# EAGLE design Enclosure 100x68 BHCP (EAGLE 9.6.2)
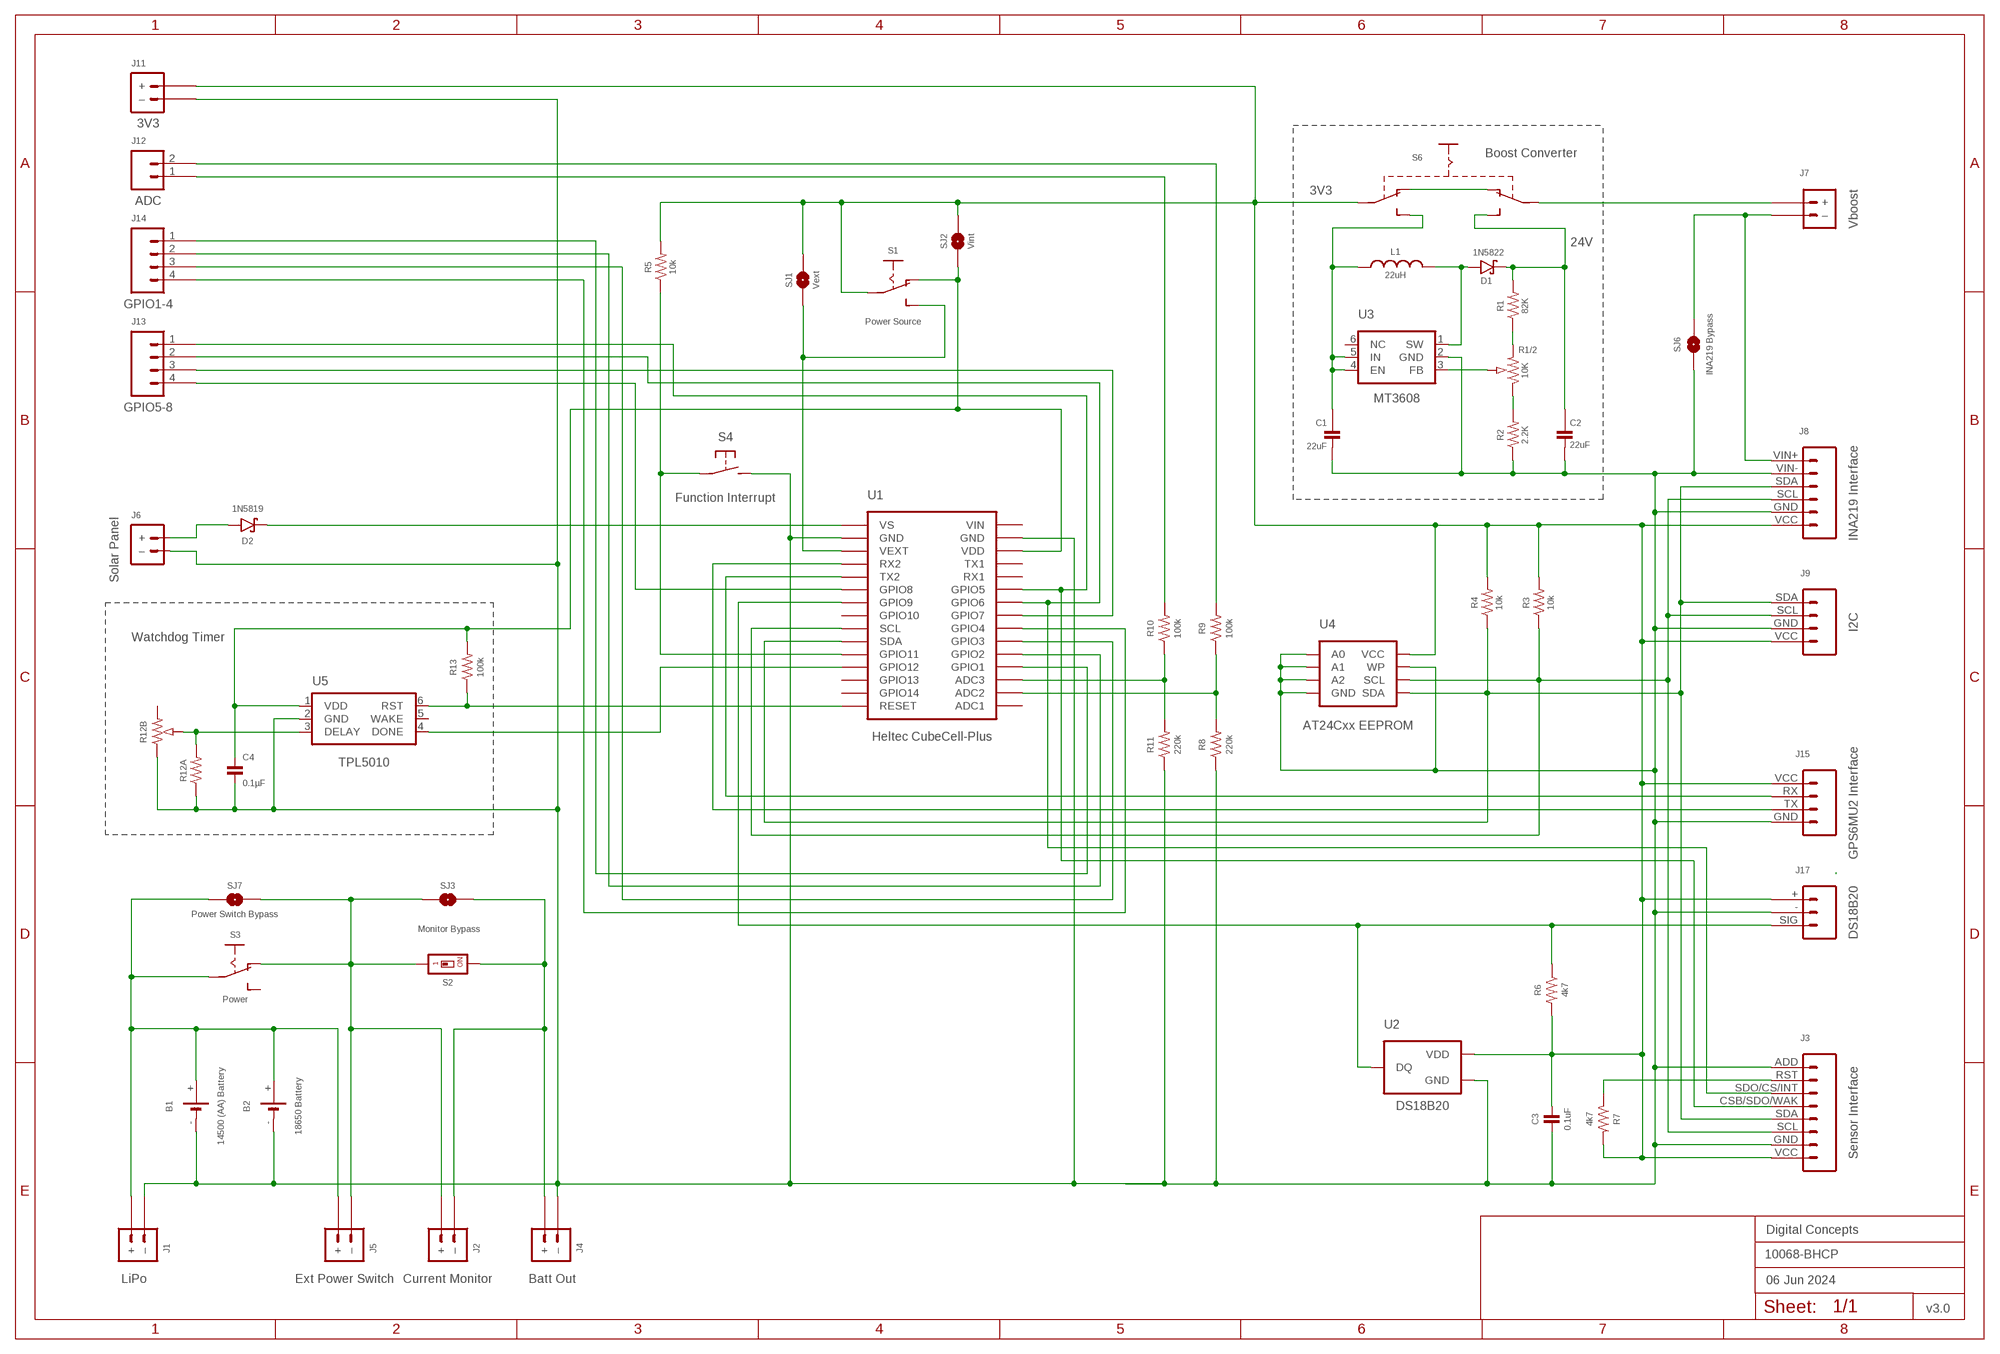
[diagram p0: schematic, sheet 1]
FRAME2 (A3L-LOC): DATE: 06 Jun 2024; OWNER: Digital Concepts; TITLE: 10068-BHCP; VERSION: v3.0

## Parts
B1  14500 (AA) Battery  BATTERY-HOLDER-14500(AA)  [BATTERY-14500]
B2  18650 Battery  BATTERY-HOLDER-18650  [BATTERY-18650]
C1  22uF  CAPACITOR-1206  [C1206]
C2  22uF  CAPACITOR-1206  [C1206]
C3  0.1uF  CAPACITOR-0805  [C0805]
C4  0.1µF  CAPACITOR-0805  [C0805]
D1  1N5822  DIODE-SCHOTTKY-1N5822  [DIODE_SMB]
D2  1N5819  1N5819-SOD-123  [SOD-123]
J1  LiPo  JST-PH2.0-2-H-POWER  [JST-PH2.0-2-HORIZONTAL-POWER]
J2  Current Monitor  JST-PH2.0-2-H-POWER  [JST-PH2.0-2-HORIZONTAL-POWER]
J3  Sensor Interface  HEADER-1X8-SENSOR  [CONN_08-SENSOR]
J4  Batt Out  JST-GH1.25-2-HORIZONTAL-POWER  [JST-GH1.25-2-HORIZONTAL]
J5  Ext Power Switch  JST-PH2.0-2-DUAL-POWER"  [JST-PH2.0-2-DUAL-POWER]
J6  Solar Panel  JST-PH2.0-2-VERTICAL  [JST-PH2.0-2-VERTICAL=POWER]
J7  Vboost  JST-PH2.0-2-H-POWER  [JST-PH2.0-2-HORIZONTAL-POWER]
J8  INA219 Interface  INA219-I2C-MODULE  [CONN_06-INA219]
J9  I2C  JST-PH2.0-I2C-MALE-HORIZONTAL  [JST-PH2.0-4-HORIZONTAL@1]
J11  3V3  JST-PH2.0-2-H-POWER  [JST-PH2.0-2-HORIZONTAL-POWER]
J12  ADC  JST-PH2.0-2-HORIZONTAL  [JST-PH2.0-2-HORIZONTAL]
J13  GPIO5-8  JST-PH2.0-4-HORIZONTAL  [JST-PH2.0-4-HORIZONTAL]
J14  GPIO1-4  JST-PH2.0-4-HORIZONTAL  [JST-PH2.0-4-HORIZONTAL]
J15  GPS6MU2 Interface  HEADER-1X4-GPS  [CONN_04-GPS]
J17  DS18B20  JST-PH2.0-3-HORIZONTAL-DS18B20  [JST-PH2.0-DS18B20-HORIZONTAL]
L1  22uH  INDUCTOR-CDRH104R/6D28L5038P  [CDRH104R+6D28]
R1  82K  RESISTORR0805  [R0805]
R1/2  10K  RESISTOR-TRIMM-BAOTER-H-US  [RTRIM64P]
R2  2.2K  RESISTORR0805  [R0805]
R3  10k  RESISTORR0805  [R0805]
R4  10k  RESISTORR0805  [R0805]
R5  10k  RESISTORR0805  [R0805]
R6  4k7  RESISTORR0805  [R0805]
R7  4k7  RESISTORR0805  [R0805]
R8  220k  RESISTORR0805  [R0805]
R9  100k  RESISTORR0805  [R0805]
R10  100k  RESISTORR0805  [R0805]
R11  220k  RESISTORR0805  [R0805]
R12A  RESISTORR0805  [R0805]
R12B  RESISTOR-TRIMM-33-US  [RTRIM3*3]
R13  100k  RESISTORR0805  [R0805]
S1  Power Source  SWITCH-SLIDE-SPDT-SMT  [SWITCH-SPDT-SMT]
S2  Monitor Bypass  SWITCH-DIP-SWS001  [SMD-001]
S3  Power  SWITCH-SLIDE-SPDT-PTH  [SWITCH-SPDT-PTH]
S4  Function Interrupt  SWITCH-MOMENTARY-2-PIN  [SWITCH-2-PAD]
S6  SWITCH-SLIDE-DPDT-PTH-S  [SWITCH-DPDT-PTH]
SJ1  Vext  SJ  [SJ]
SJ2  Vint  SJ-V-12  [SJ-VIA-12]
SJ3  Monitor  SJ  [SJ]
SJ6  INA219 Bypass  SJ  [SJ]
SJ7  Power Switch Bypass  SJ  [SJ]
U1  Heltec CubeCell-Plus  HELTEC-CUBECELL-PLUS-X  [HELTEC-CUBECELL=PLUS-X]
U2  DS18B20  THERMOMETER-DS18B20  [TO-92]
U3  MT3608  [SOT-23-6]
U4  AT24Cxx EEPROM  AT24CXX-EEPROM  [SOP-8]
U5  TPL5010  TPL5010DDCR  [SOT-23-6]

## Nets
GND: B1.- B2.- C1.2 C2.2 C3.2 C4.2 J1.-(–) J3.ADD J3.GND J4.-(–) J6.-(–) J8.GND J8.VIN- J9.GND J11.-(–) J15.GND J17.- R2.1 R8.1 R11.1 R12A.1 R12B.1(A) S4.P$2(S) SJ6.1 U1.GND@14(GND) U1.GND@17(GND) U2.1(GND) U3.2(GND) U4.P$1(A0) U4.P$2(A1) U4.P$3(A2) U4.P$4(GND) U4.P$7(WP) U5.2(GND)
N$1: D2.A J6.+
N$2: R10.1 R11.2 U1.ADC3
N$3: J2.-(–) J4.+ S2.2 SJ3.1
N$4: B1.+ B2.+ J1.+ J5.+ S3.2(P) SJ7.2
N$5: D2.C U1.VS
N$6: D1.A L1.1 U3.1(SW)
N$7: J12.1 R10.2
N$8: J3.SCL J8.SCL J9.SCL R3.1 U1.SCL U4.P$6(SCL)
N$9: J3.RST R7.1
N$10: J3.CSB/SDO/WAK J13.1 U1.GPIO5
N$11: J3.SDA J8.SDA J9.SDA R4.1 U1.SDA U4.P$5(SDA)
N$12: J13.4 U1.GPIO8
N$13: S1.3(S) SJ1.1 U1.VEXT
N$14: J15.RX U1.TX2
N$15: J7.-(–) J8.VIN+ SJ6.2
N$16: J15.TX U1.RX2
N$18: R12A.2 R12B.2(S) U5.3(DELAY)
N$19: J3.SDO/CS/INT J13.2 U1.GPIO6
N$20: J7.+ S6.P$2(P1)
N$21: J2.+ J5.-(–) S2.1 S3.1(O) SJ3.2 SJ7.1
N$22: R1/2.2(S) U3.3(FB)
N$23: R1/2.1(A) R2.2
N$24: J17.SIG R6.1 U1.GPIO9 U2.2(DQ)
N$25: C1.1 L1.2 S6.P$6(S2) U3.4(EN) U3.5(IN)
N$26: S6.P$1(O1) S6.P$4(O2)
N$27: R5.1 S4.P$1(P) U1.GPIO11
N$28: C2.1 D1.C R1.2 S6.P$3(S1)
N$29: J14.1 U1.GPIO1
N$30: J14.2 U1.GPIO2
N$32: J12.2 R9.2
N$33: R8.2 R9.1 U1.ADC2
N$34: R13.1 U1.RST(RESET) U5.6(RST)
N$35: J14.3 U1.GPIO3
N$36: J14.4 U1.GPIO4
N$37: U1.GPIO12 U5.4(DONE)
N$38: R1.1 R1/2.3(E)
N$39: C4.1 R13.2 S1.1(O) SJ2.1 SJ2.1@V U1.VDD U5.1(VDD)
N$40: J13.3 U1.GPIO7
VEXT: C3.1 J3.VCC J8.VCC J9.VCC J11.+ J15.VCC J17.+ R3.2 R4.2 R5.2 R6.2 R7.2 S1.2(P) S6.P$5(P2) SJ1.2 SJ2.2 SJ2.2@V U2.3(VDD) U4.P$8(VCC)
Unconnected: R12B.3(E) S3.3(S) U1.ADC1 U1.GPIO10 U1.GPIO13 U1.GPIO14 U1.RX1 U1.TX1 U3.6(NC) U5.5(WAKE)

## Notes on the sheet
- Boost Converter
- 3V3
- 24V
- Watchdog Timer

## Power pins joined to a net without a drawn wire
VIN: U1.VIN

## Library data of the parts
B1 = digitalconcepts:BATTERY-HOLDER-14500(AA): 14500 (AA) battery holder
B2 = digitalconcepts:BATTERY-HOLDER-18650: 18650 Battery Holder
C1 C2 = digitalconcepts:CAPACITOR-1206: 1206 Capacitor
C3 C4 = digitalconcepts:CAPACITOR-0805: 0805 Capacitor
D1 = digitalconcepts:DIODE-SCHOTTKY-1N5822: 1N5822 Schottky Diode SMB
D2 = digitalconcepts:1N5819-SOD-123: 1N5819 Schottky Diode SOD-123
J1 J2 J7 J11 = digitalconcepts:JST-PH2.0-2-H-POWER: PH2.0 2P Right Angle Connector with power pin labelling
J3 = digitalconcepts:HEADER-1X8-SENSOR: IoT Sensors 1x8 Pin Header for 'Sandwich' IoT Sensors
J4 = digitalconcepts:JST-GH1.25-2-HORIZONTAL-POWER: JST GH1.25 2P PTH Connector (Power)
J5 = digitalconcepts:JST-PH2.0-2-DUAL-POWER: PH2.0 2P PTH Dual-Side Connector (Power); PROD_ID: CONN-09863; SKU: PRT-09914
J6 = digitalconcepts:JST-PH2.0-2-VERTICAL: PH2.0 2P PCB Connector
J8 = digitalconcepts:INA219-I2C-MODULE: INA219 I2C Module
J9 = digitalconcepts:JST-PH2.0-I2C-MALE-HORIZONTAL: PH2.0 4P (I2C) Right Angle PCB Connector
J12 = digitalconcepts:JST-PH2.0-2-HORIZONTAL: PH2.0 2P Right Angle Connector
J13 J14 = digitalconcepts:JST-PH2.0-4-HORIZONTAL: PH2.0 4P Horizontal Connector
J15 = digitalconcepts:HEADER-1X4-GPS: NEO GPS 4-Pin Header
J17 = digitalconcepts:JST-PH2.0-3-HORIZONTAL-DS18B20: DS18B20 PH2.0 Right Angle PCB Connector
L1 = digitalconcepts:INDUCTOR-CDRH104R/6D28: Inductor; SPICEPREFIX: L
R1-R11 R12A R13 = digitalconcepts:RESISTOR: Resistor; SPICEPREFIX: R
R1/2 = digitalconcepts:RESISTOR-TRIMM-BAOTER-H-US: Trimm Resistor - Horizontal BAOTER
R12B = digitalconcepts:RESISTOR-TRIMM-3*3-US: Trimm Resistor - 3*3 SMD
S1 = digitalconcepts:SWITCH-SLIDE-SPDT-SMT: Mini Sliding Switch SPDT SMT
S2 = digitalconcepts:SWITCH-DIP-SWS001: SMD Dip Switch 1 pol.
S3 = digitalconcepts:SWITCH-SLIDE-SPDT-PTH: Mini Sliding Switch SPDT PTH
S4 = digitalconcepts:SWITCH-MOMENTARY-2-PIN: 2 Pin Momentary Switch
S6 = digitalconcepts:SWITCH-SLIDE-DPDT-PTH-S: Switch DPDT PTH-S
SJ1 SJ3 SJ6 SJ7 = digitalconcepts:SJ: Solder Jumper
SJ2 = digitalconcepts:SJ-V-12: Solder Jumper with Pad Vias
U1 = digitalconcepts:HELTEC-CUBECELL-PLUS-X: Heltec CubeCell Dev-Board Plus Excluding internal pins
U2 = digitalconcepts:THERMOMETER-DS18B20: Digital Thermometer -55C-125C TO92-3; AVAILABILITY: Bad; DESCRIPTION: Temperature Sensor Digital, Local -55°C ~ 125°C 12 b 8-uMAX; MF: Maxim Integrated; MP: DS18B20; PACKAGE: TO-92 Maxim Integrated; PRICE: None
U3 = digitalconcepts:MT3608: MT3608 DC-DC Step-Up Voltage Converter
U4 = digitalconcepts:AT24CXX-EEPROM: AT24Cxx EEPROM SOP-8
U5 = digitalconcepts:TPL5010DDCR: TPL5010 Nano-Power System Timer with Watchdog

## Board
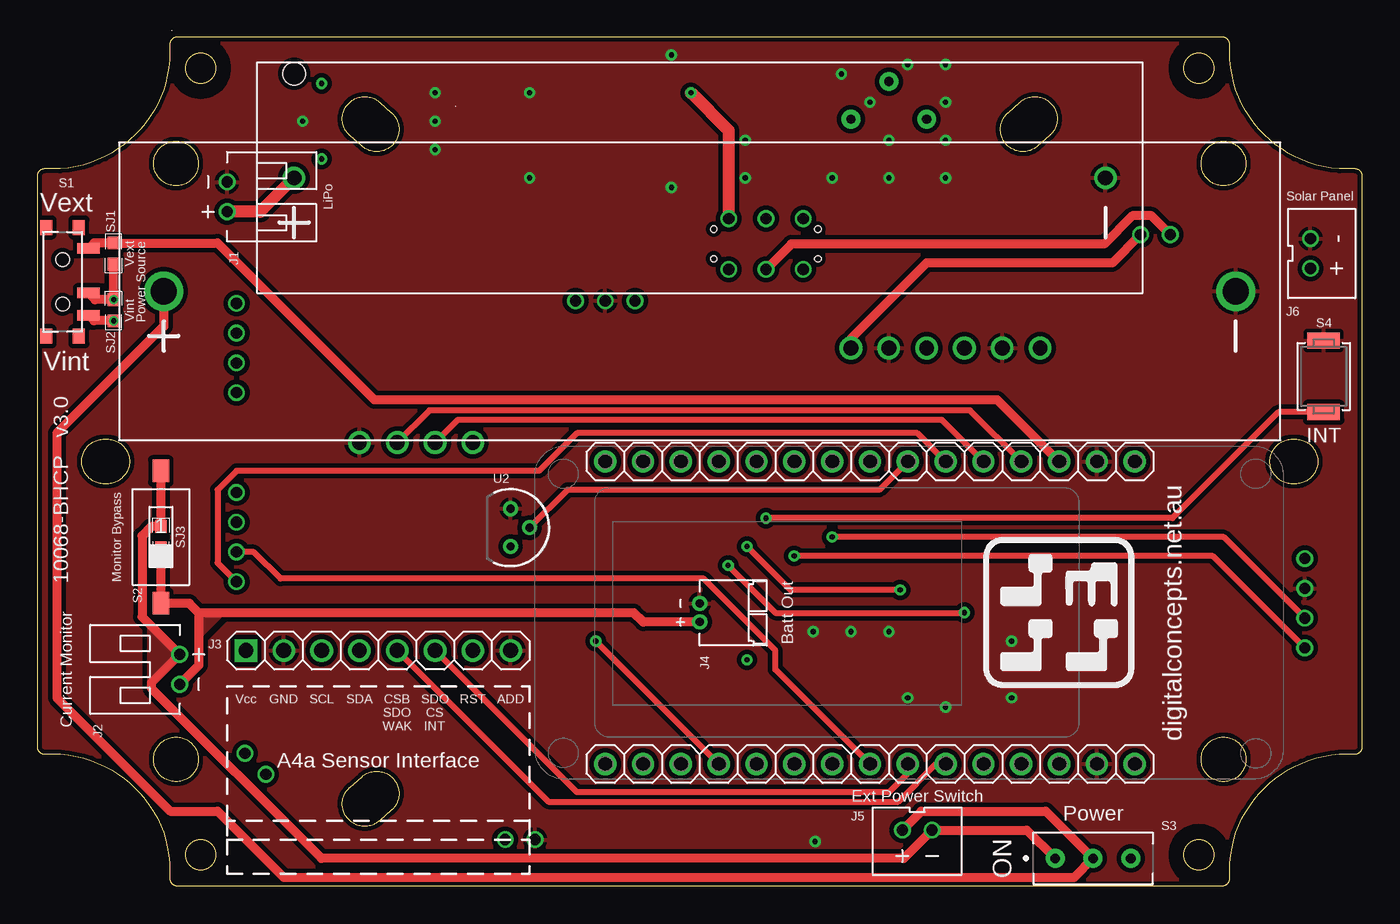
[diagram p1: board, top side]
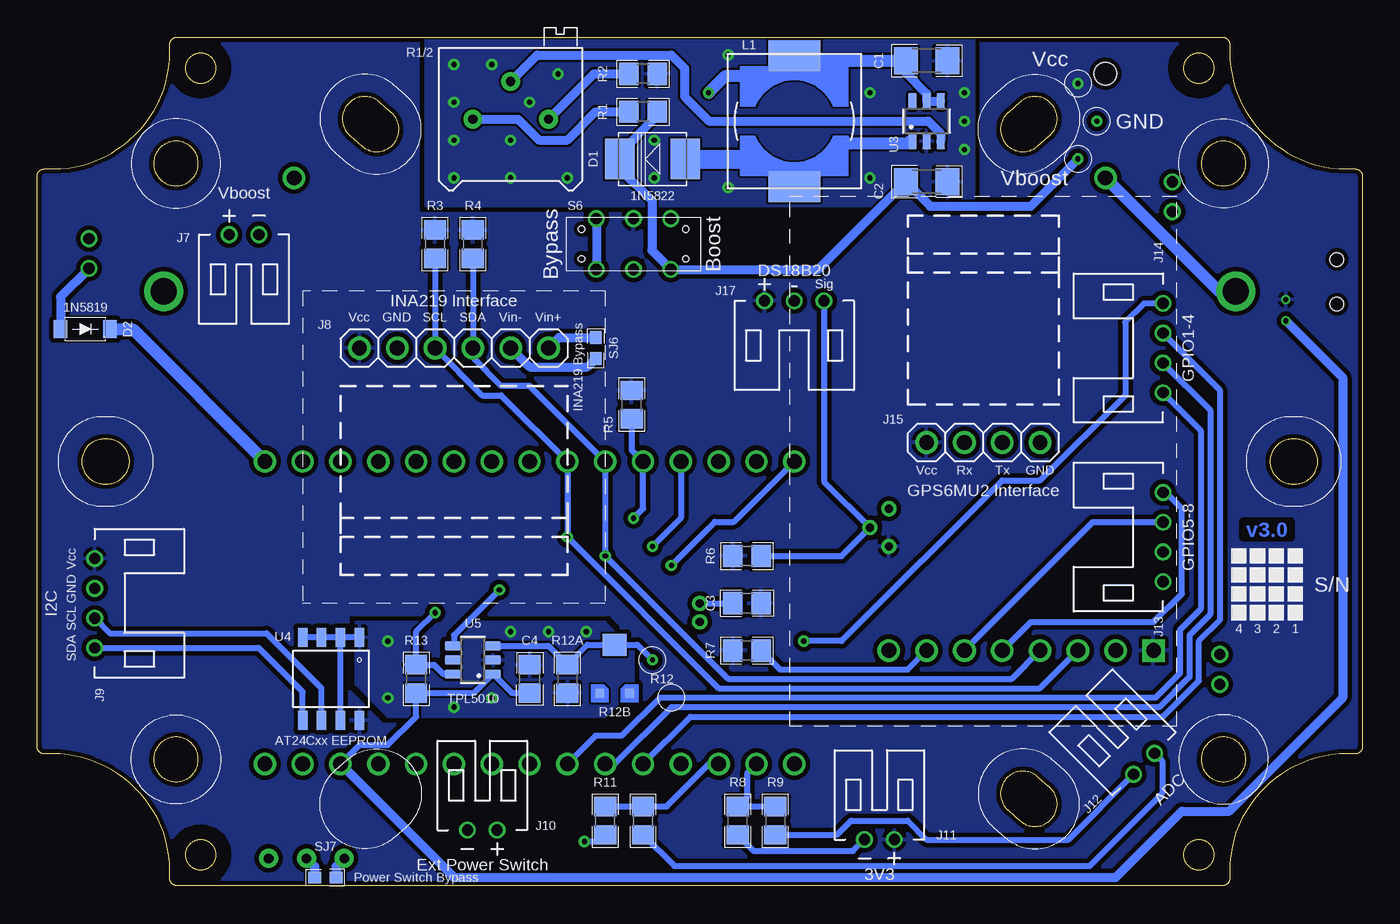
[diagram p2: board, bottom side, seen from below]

Size 89 x 57 mm. Coordinates in mm from the lower left corner, seen from the top.
Outline: 1134 segments
Outline: circle at 10.97,2.08 radius 1.02
Outline: circle at 10.97,54.92 radius 1.02
Outline: circle at 78.03,54.92 radius 1.02
Outline: circle at 78.03,2.08 radius 1.02
Copper layers (1*16): Top 0.035mm / dielectric 1.5mm / Bottom 0.035mm
Design rules "default *": minimum track width 6mil, minimum drill 0.35mm, track to track 6mil, track to pad 6mil, pad to pad 6mil, via to via 6mil, smd to smd 6mil, copper to edge 6mil, drill to drill 6mil, minimum pad ring 1mil, minimum via ring 8mil, stop-mask expansion 4mil, vias tented up to drill 0mil, thermal gap 10mil

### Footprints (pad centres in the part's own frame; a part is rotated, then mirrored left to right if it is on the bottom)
BATTERY-14500 = drill 1: + -27.25,0; - 27.25,0 | hole 1.524: -27.25,7
BATTERY-18650 = drill 1.75: + -36,0; - 36,0
C1206 = smd 1.6 x 1.8: 1 -1.4,0; 2 1.4,0
C0805 = smd 1.3 x 1.5: 1 -0.95,0; 2 0.95,0
DIODE_SMB = smd 2 x 2.7: A 2.2,0; C -2.2,0
SOD-123 = smd 0.91 x 1.22: A -1.65,0; C 1.65,0
JST-PH2.0-2-HORIZONTAL-POWER = drill 0.75: + 1,0; - -1,0
CONN_08-SENSOR = drill 1 pad 1.524: ADD 17.78,0; CSB/SDO/WAK 10.16,0; GND 2.54,0; RST 15.24,0; SCL 5.08,0; SDA 7.62,0; SDO/CS/INT 12.7,0 | drill 1 pad 1.524 square: VCC 0,0
JST-GH1.25-2-HORIZONTAL = drill 0.55 pad 1.016: + -0.625,0; - 0.625,0
JST-PH2.0-2-DUAL-POWER = drill 0.75: + 1,0; - -1,0
JST-PH2.0-2-VERTICAL=POWER = drill 0.75: + -1,0; - 1,0
CONN_06-INA219 = drill 1 pad 1.524: GND 2.54,0; SCL 5.08,0; SDA 7.62,0; VCC 0,0; VIN+ 12.7,0; VIN- 10.16,0
JST-PH2.0-4-HORIZONTAL@1 = drill 0.75: GND -1,0; SCL 1,0; SDA 3,0; VCC -3,0
JST-PH2.0-2-HORIZONTAL = drill 0.75: 1 1,0; 2 -1,0
JST-PH2.0-4-HORIZONTAL = drill 0.75: 1 3,0; 2 1,0; 3 -1,0; 4 -3,0
CONN_04-GPS = drill 1 pad 1.524: GND 0,0; RX 5.08,0; TX 2.54,0; VCC 7.62,0
JST-PH2.0-DS18B20-HORIZONTAL = drill 0.75: + 2,0; - 0,0; SIG -2,0
CDRH104R+6D28 = smd 2.1 x 3.5: 1 -4.4,0; 2 4.4,0
R0805 = smd 1.3 x 1.5: 1 -0.95,0; 2 0.95,0
RTRIM64P = drill 0.61 pad 1.27: 1 0,-2.54; 2 2.54,0; 3 0,2.54
RTRIM3*3 = smd 0.6 x 0.6: 1 -1,-1.6; 3 1,-1.6 | smd 1.6 x 1.5: 2 0,1.65
SWITCH-SPDT-SMT = smd 0.7 x 1.5: 1 2.25,1.75; 2 0.75,1.75; 3 -2.25,1.75 | smd 1 x 0.8: GND@1 3.65,-1.1; GND@2 3.65,1.1; GND@3 -3.65,1.1; GND@4 -3.65,-1.1 | hole 0.9: -1.5,0; 1.5,0
SMD-001 = smd 1.1 x 1.5: 1 0,-4.45; 2 0,4.45
SWITCH-SPDT-PTH = drill 0.65 pad 1.27: 1 -2.54,0; 2 0,0; 3 2.54,0
SWITCH-2-PAD = smd 1.067 x 2.184: P$1 -2.4,0; P$2 2.4,0
SWITCH-DPDT-PTH = drill 0.75: P$1 -1.7,2.5; P$2 -1.7,0; P$3 -1.7,-2.5; P$4 1.7,2.5; P$5 1.7,0; P$6 1.7,-2.5 | hole 0.42: 1,3.5; -1,3.5; 1,-3.5; -1,-3.5
SJ = smd 0.864 x 0.762: 1 -0.711,0; 2 0.711,0
SJ-VIA-12 = smd 0.864 x 0.762: 1 -0.711,0; 2 0.711,0 | drill 0.35 pad 0.61: 1@V -0.711,0; 2@V 0.711,0
HELTEC-CUBECELL=PLUS-X = drill 1: ADC1 0,0; ADC2 0,2.54; ADC3 0,5.08; GND@14 0,33.02; GND@17 -20.32,33.02; GPIO1 0,7.62; GPIO2 0,10.16; GPIO3 0,12.7; GPIO4 0,15.24; GPIO5 0,22.86; GPIO6 0,20.32; GPIO7 0,17.78; GPIO8 -20.32,22.86; GPIO9 -20.32,20.32; GPIO10 -20.32,17.78; GPIO11 -20.32,10.16; GPIO12 -20.32,7.62; GPIO13 -20.32,5.08; GPIO14 -20.32,2.54; RST -20.32,0; RX1 0,25.4; RX2 -20.32,27.94; SCL -20.32,15.24; SDA -20.32,12.7; TX1 0,27.94; TX2 -20.32,25.4; VDD 0,30.48; VEXT -20.32,30.48; VIN 0,35.56; VS -20.32,35.56
TO-92 = drill 0.55 pad 1.016: 1 -1.27,0; 2 0,1.27; 3 1.27,0
SOT-23-6 = smd 1.1 x 0.6: 1 -1.35,0.95; 2 -1.35,0; 3 -1.35,-0.95; 4 1.35,-0.95; 5 1.35,0; 6 1.35,0.95
SOP-8 = smd 0.635 x 1.27: P$1 -1.905,-2.794; P$2 -0.635,-2.794; P$3 0.635,-2.794; P$4 1.905,-2.794; P$5 1.905,2.794; P$6 0.635,2.794; P$7 -0.635,2.794; P$8 -1.905,2.794

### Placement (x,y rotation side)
B1  44.5,47.55 0 top
B2  44.5,39.93 0 top
C1  29.26,55.42 0 bottom
C2  29.26,47.3 0 bottom
C3  41.32,18.97 180 bottom
C4  55.93,13.89 90 bottom
D1  47.67,48.82 0 bottom
D2  85.77,37.39 0 bottom
J1  12.75,46.28 270 top
J2  9.57,14.53 90 top
J3  14.02,15.8 0 top
J4  44.5,18.34 90 top
J5  59.1,3.73 0 bottom
J6  85.52,42.47 90 top
J7  75.11,43.74 180 bottom
J8  67.36,36.12 0 bottom
J9  85.14,18.97 270 bottom
J11  32.43,3.1 0 bottom
J12  14.65,8.18 45 bottom
J13  13.38,23.42 90 bottom
J14  13.38,36.12 90 bottom
J15  21.64,29.77 180 bottom
J17  38.15,39.29 180 bottom
L1  38.15,51.36 90 bottom
R1  48.31,51.99 0 bottom
R1/2  57.2,51.49 90 bottom
R2  48.31,54.53 180 bottom
R3  62.28,43.1 90 bottom
R4  59.74,43.1 90 bottom
R5  49.07,32.31 90 bottom
R6  41.32,22.15 180 bottom
R7  41.32,15.8 180 bottom
R8  41.96,4.37 90 bottom
R9  39.42,4.37 270 bottom
R10  48.31,4.37 270 bottom
R11  50.85,4.37 90 bottom
R12A  53.39,13.89 90 bottom
R12B  50.21,14.53 0 bottom
R13  63.55,13.89 270 bottom
S1  1.7,40.56 270 top
S2  8.3,23.42 180 top
S3  70.92,1.83 0 top
S4  86.41,34.21 90 top
S6  48.94,43.1 90 bottom
SJ1  5.13,42.47 270 top
SJ2  5.13,38.66 90 top
SJ3  8.3,23.42 90 top
SJ6  51.48,36.12 90 bottom
SJ7  69.65,0.56 180 bottom
U1  38.15,8.18 270 top
U2  31.8,24.05 270 top
U3  29.26,51.36 90 bottom
U4  69.26,13.89 180 bottom
U5  59.74,15.16 180 bottom

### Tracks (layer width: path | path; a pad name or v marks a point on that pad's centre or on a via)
$X
  cutout Bottom: 10.97,56.95 arc180 10.97,52.88 arc180
$X1
  cutout Bottom: 78.03,56.95 arc180 78.03,52.88 arc180
$X2
  cutout Top: 78.03,4.12 arc180 78.03,0.05 arc180
$X3
  cutout Top: 10.97,4.12 arc180 10.97,0.05 arc180
$X4
  cutout Top: 10.97,56.95 arc180 10.97,52.88 arc180
$X5
  cutout Top: 78.03,56.95 arc180 78.03,52.88 arc180
$X6
  cutout Bottom: 78.03,4.12 arc180 78.03,0.05 arc180
$X7
  cutout Bottom: 10.97,4.12 arc180 10.97,0.05 arc180
GND  (via drill 0.35)
  Bottom 0.406: R11.1 51.3,2.97 v52.25,2.97 | J4.- C3.2 | U4.P$7 U4.P$2 | U4.P$1 U4.P$2 | U4.P$2 U4.P$3 U4.P$4 | R12B.1 50.86,12.93 | R8.1 40.88,2.34 34.2,2.34 J11.-
  Bottom 0.61: J8.VIN- 55.93,34.85 52.04,34.85 SJ6.1
  other vias: 26.72,53.26 58.47,55.17 54.02,54.53 47.55,50.09 47.55,47.55 53.39,47.55 57.2,47.55 57.2,50.09 61.01,47.55 61.01,50.09 61.01,55.17 26.72,51.36 55.93,52.63 61.01,52.63 42.59,46.91 42.59,55.8 33.07,53.26 33.07,47.55 26.72,49.45 17.83,51.36 52.12,17.07 54.66,17.07 57.2,17.07 65.45,16.43 65.45,12.62 61.01,11.99 58.47,12.62
  pour Top (isolate 0.305, rank 2): -1.65,58.87 -1.65,-1.92 90.59,-1.92 90.59,58.87
  pour Bottom: 26.08,57.07 26.08,45.64 62.91,45.64 62.91,57.07
  pour Bottom: 67.61,17.7 67.61,13.51 65.45,11.35 50.85,11.35 48.94,13.26 48.94,15.8 50.85,17.7
N$1
  Bottom 0.61: J6.+ 87.42,39.57 D2.A
N$2
  Bottom 0.406: R11.2 R10.1 46.72,5.32 43.86,8.18 U1.ADC3
N$3
  Top 0.61: SJ3.1 S2.2 10.21,18.97 10.84,18.34 | J2.- 10.84,14.8 10.84,18.34 | J4.+ 40.69,17.71 40.06,18.34 10.84,18.34
  pour Top: 10.84,18.34 10.84,16.56 12.62,18.34
N$4
  Top 0.61: J5.+ 59.37,5 67.74,5 S3.2 69.65,0.56 16.56,0.56 12.11,5 8.94,5 1.32,12.62 1.32,30.4 8.5,37.58 B2.+
  Top 0.813: B1.+ 14.98,45.28 J1.+
  Bottom 0.61: S3.2 70.36,1.27 SJ7.2
  Bottom 0.813: B1.+ 9.63,39.93 B2.+
N$5
  Bottom 0.813: D2.C 82.6,37.39 U1.VS
N$6
  Bottom 0.152: U3.1 30.4,50.01
  Bottom 0.406: 40.5,48.82 38.64,46.96 L1.1 37.96,46.96 35.04,49.88
  Bottom 0.813: 35.04,49.88 30.53,49.88 30.4,50.01
  Bottom 1.27: D1.A 40.5,48.82
N$7
  Bottom 0.406: R10.2 46.21,1.32 18.31,1.32 13.44,6.19 13.44,8.38 J12.1
N$8  (via drill 0.35)
  Top 0.406: J9.SCL 79.69,23.42 v53.39,23.42
  Bottom 0.406: J3.SCL 21.64,13.26 43.23,13.26 v53.39,23.42 U1.SCL 57.83,32.94 59.1,32.94 J8.SCL R3.1 | U4.P$6 69.9,13.26 73.6,16.96 84.12,16.96 J9.SCL
N$9
  Bottom 0.406: R7.1 39.1,14.53 30.53,14.53 J3.RST
N$10
  Top 0.406: J3.CSB/SDO/WAK 34.34,5.64 57.83,5.64 60.37,8.18 U1.GPIO5
  Bottom 0.406: J3.CSB/SDO/WAK 22.27,17.7 14.02,17.7 12.11,19.61 12.11,25.32 13.21,26.42 J13.1
N$11  (via drill 0.35)
  Top 0.406: J9.SDA 78.95,22.15 v50.85,22.15
  Bottom 0.406: J3.SDA 23.54,13.89 42.59,13.89 v50.85,22.15 U1.SDA 55.93,33.58 57.83,33.58 59.74,35.48 J8.SDA R4.1 | J9.SDA 74.14,15.97 71.17,13.01 U4.P$5
N$12
  Top 0.406: U1.GPIO8 59.1,30.4 36.24,30.4 33.7,27.86 13.38,27.86 12.11,26.59 12.11,21.69 J13.4
N$13
  Top 0.61: U1.VEXT 64.49,32.64 22.66,32.64 12.11,43.18 SJ1.1 3.82,43.18 S1.3
N$14
  Top 0.406: J15.RX 28.24,31.29 60.76,31.29 U1.TX2
N$15
  Top 0.61: J7.- 72.2,41.83 59.74,41.83 54.66,36.75 J8.VIN+
  Bottom 0.61: J8.VIN+ 53.95,36.83 SJ6.2
N$16
  Top 0.406: J15.TX 26.34,31.93 62.66,31.93 U1.RX2
N$18  (via drill 0.35)
  Bottom 0.406: U5.3 54.66,16.11 R12A.2 52.05,16.18 R12B.2 48.69,16.18 v47.67,15.16
N$19
  Top 0.406: J3.SDO/CS/INT 36.24,6.27 57.2,6.27 58.47,7.54 U1.GPIO6
  Bottom 0.406: J3.SDO/CS/INT 18.1,24.42 J13.2
N$20
  Top 0.61: J7.+ 74.84,45.01 73.57,45.01 71.66,43.1 50.64,43.1 S6.P$2
N$21
  Top 0.61: S2.1 SJ3.2 7.67,24.13 7.03,23.5 7.03,18.07 J2.+ 7.67,13.62 7.67,13.26 19.1,1.83 58.2,1.83 J5.- 66.47,3.73 S3.1
  Bottom 0.61: S3.1 68.93,1.27 SJ7.1
  pour Top (no thermals): 9.57,15.53 7.67,17.43 7.67,13.62
N$22
  Bottom 0.61: U3.3 28.31,50.51 29.16,51.36 43.86,51.36 45.52,53.01 45.52,54.92 46.4,55.8 55.42,55.8 R1/2.2
N$23
  Bottom 0.61: R1/2.1 51.61,54.53 R2.2
N$24
  Top 0.406: U1.GPIO9 56.56,26.59 35.61,26.59 U2.2
  Bottom 0.406: R6.1 34.97,22.15 U2.2 36.15,27.13 J17.SIG
N$25  (via drill 0.35)
  Top 0.813: v43.9,53.26 46.44,50.72 S6.P$6
  Bottom 0.61: C1.1 30.66,54.61 29.26,53.21 U3.5 U3.4
  Bottom 0.813: C1.1 37.68,55.42 L1.2 38.53,55.76 39.88,54.41 42.76,54.41 v43.9,53.26
N$26
  Bottom 0.61: S6.P$4 S6.P$1
N$27  (via drill 0.35)
  Top 0.406: S4.P$1 83.37,31.81 76.25,24.69 v48.94,24.69
  Bottom 0.406: v48.94,24.69 48.31,25.32 U1.GPIO11 49.07,29.26 R5.1
N$28  (via drill 0.35)
  Bottom 0.61: v19.1,48.82 22.27,45.64 29.01,45.64 C2.1 36.55,41.4 S6.P$3 47.71,42.67 47.71,46.02 49.87,48.18 D1.C 50,48.95 50,49.07 47.36,51.71 R1.2
N$29  (via drill 0.35)
  Top 0.406: v37.51,16.43 U1.GPIO1
  Bottom 0.406: J14.1 14.65,39.12 15.92,37.85 15.92,32.94 21.64,27.23 24.18,27.23 34.97,16.43 v37.51,16.43
N$30
  Bottom 0.406: J14.2 9.57,33.31 9.57,17.83 10.97,16.43 10.97,13.77 13.38,11.35 45.13,11.35 U1.GPIO2
N$32
  Bottom 0.406: R9.2 35.29,3.42 34.34,4.37 30.53,4.37 29.26,3.1 19.73,3.1 J12.2
N$33
  Bottom 0.406: R9.1 R8.2 41.32,5.95 41.32,7.54 U1.ADC2
N$34  (via drill 0.35)
  Top 0.406: v46.4,21.51 49.58,18.34 v62.28,18.34
  Bottom 0.406: U5.6 61.72,14.21 62.36,14.85 64.18,14.85 64.17,14.84 R13.1 63.55,17.07 v62.28,18.34 | U1.RST 42.21,24.44 43.48,24.44 v46.4,21.51
N$35
  Bottom 0.406: J14.3 10.21,31.94 10.21,18.21 11.61,16.82 11.61,14.02 13.64,11.99 46.4,11.99 50.21,8.18 U1.GPIO3
N$36
  Bottom 0.406: J14.4 10.84,30.58 10.84,18.59 12.24,17.2 12.24,14.28 13.89,12.62 47.18,12.62 49.74,10.07 51.5,10.07 U1.GPIO4
N$37  (via drill 0.35)
  Top 0.406: v47.67,22.78 50.6,19.86 v57.96,19.86
  Bottom 0.406: U5.4 61.01,16.19 61.01,16.82 v57.96,19.86 | U1.GPIO12 45.77,24.69 v47.67,22.78
N$38
  Bottom 0.61: R1/2.3 56.69,51.49 55.29,50.09 53.39,50.09 51.48,51.99 R1.1
N$39
  Top 0.61: SJ2.1@V 3.82,37.95 S1.1
  Bottom 0.406: C4.1 57.12,12.94 U5.1 59.66,12.94 R13.2 63.55,11.35 65.45,9.45 67.36,9.45 U1.VDD
  Bottom 0.61: U1.VDD 61.01,0.56 16.56,0.56 12.11,5 8.94,5 1.32,12.62 1.32,34.14 SJ2.1@V
N$40
  Top 0.406: J13.3 14.54,22.42 16.34,20.63 44.75,20.63 49.58,15.8 49.58,14.53 U1.GPIO7
VEXT  (via drill 0.35)
  Top 0.61: S1.2 3.89,39.37 SJ2.2@V SJ1.2
  other vias: 19.1,53.9
  pour Bottom (isolate 0.305, rank 2): -0.65,57.87 -0.65,-0.92 89.59,-0.92 89.59,57.87

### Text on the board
Bottom: v3.0
tPlace: 10068-BHCP v3.0 | digitalconcepts.net.au | Vcc | GND | SCL | SDA | RST | ADD | CSB / SDO / WAK | SDO / CS / INT
bPlace: Vin+ | Vin- | SDA | SCL | GND | Vcc | GND | Tx | Rx | Vcc | S/N | 1 | 2 | 3 | 4
tNames: Vext | Vint | INT | A4a Sensor Interface | ON
bNames: Vcc | GND | Vboost | Boost | Bypass | Vcc | GND | SCL | SDA | R12 | J10 | Ext Power Switch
